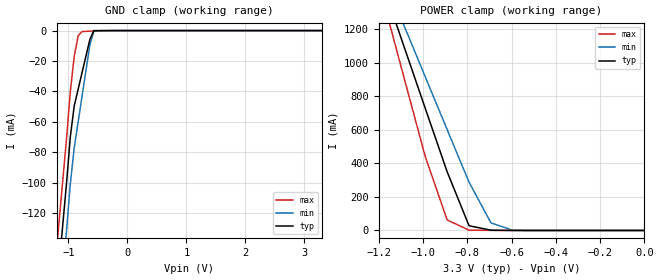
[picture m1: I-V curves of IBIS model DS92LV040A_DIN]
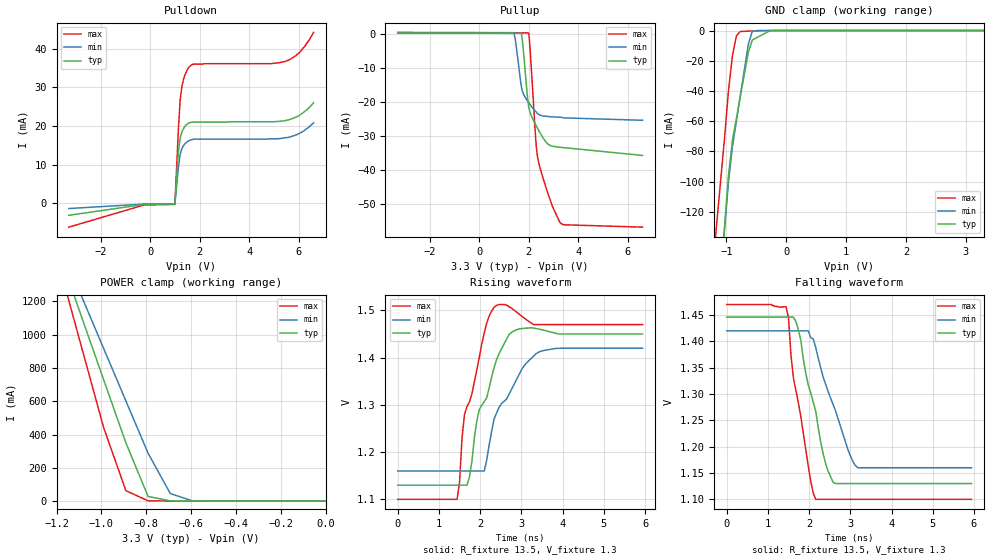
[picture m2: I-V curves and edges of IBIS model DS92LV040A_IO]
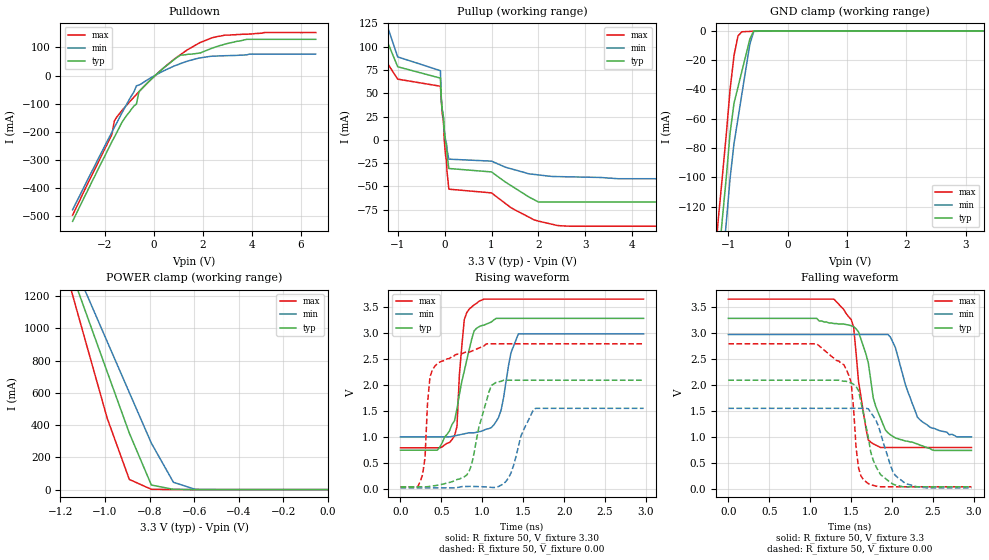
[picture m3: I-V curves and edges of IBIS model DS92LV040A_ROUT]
|   National Semiconductor Corporation
|   IBIS Model of DS92LV040A
|   4 Channel Bus LVDS Transceiver
|   44 Lead LLP Package
[IBIS Ver]   3.2
[Comment Char]   |_char
[File name]   ds92lv040atlqa.ibs
[File Rev]   2.2
[Date]   08/23/04
[Source]
SPICE to IBIS Translation
[Notes]
Created by Tim Coyle
Rev2.1 adjusted IOM and IOP rise fall tables for monotonicity--milt
Rev2.2 Updated Power clamp tables, C-comp, Pin, Package, and Ramp;
   New DS92LV040A_IO model; dglisic
[Disclaimer]
(C) Copyright National Semiconductor Corporation 2002
   All rights reserved
   National Semiconductor Corporation hereby grants
the user of this IBIS model a non-exclusive, nontransferable
license to use this IBIS model under the following terms.
Before using this IBIS model, the user should read this
license.  If the user does not accept these terms,  the
IBIS model should be returned to National within 30 days.
   The user is granted this license only to use the
IBIS model and is not granted rights to sell, load, rent,
lease or license the IBIS model in whole or in part, or in
modified form to anyone other than user. User may modify
the IBIS model to suit its specific applications but rights
to derivative works and such modifications shall belong to
National.
   This IBIS model is provided on an "AS IS" basis and
National makes absolutely no warranty with respect to the
information contained herein.NATIONAL DISCLAIMS AND CUSTOMER
WAIVES ALL WARRANTIES, EXPRESS OR IMPLIED, INCLUDING
WARRANTIES OF MERCHANTABILITY OR FITNESS FOR A PARTICULAR
PURPOSE. The entire risk as to quality and performance is
with the Customer. ACCORDINGLY, IN NO EVENT SHALL THE
COMPANY BE LIABLE FOR ANY DAMAGES, WHETHER IN CONTRACT OR
TORT,INCLUDING ANY LOST PROFITS OR OTHER INCIDENTAL,
CONSEQUENTIAL, EXEMPLARY, OR PUNITIVE DAMAGES ARISING OUT
OF THE USE OR APPLICATION OF THE IBIS model provided in
this package.Further, National reserves the right to make
changes without notice to any product herein to improve
reliability, function, or design. National does not convey
any license under patent rights or any other intellectual
property rights, including those of third parties.
   National is not obligated to provide maintenance or support
for the licensed IBIS model.
Contact National at ATTN:INTERFACE APPLICATIONS/IBIS MODELS.
5 Foden Road, M/S 03-03, South Porltand, ME 04106
(207) 541-6031
[Copyright]
(c) Copyright 2002 National Semiconductor Corp.
[Component]   DS92LV040ATLQA
Si_location Pin
Timing_location Pin
[Manufacturer]   National Semiconductor Corp.
[Package]
|   TYP   MIN   MAX
R_pkg   0.194   0.174   0.249
L_pkg   1.88n   1.46n   2.21n
C_pkg   0.084p   0.063p   0.111p
[Pin]   signal_name   model_name   R_pin   L_pin   C_pin
1   NC   NC   0.239   2.15n   0.094p
2   NC   NC   0.223   1.96n   0.074p
3   VCC   POWER   0.210   1.83n   0.071p
4   GND   GND   0.214   1.78n   0.102p
5   RE2*   DS92LV040A_CONTROL  0.222   1.80n   0.103p
6   VCC   POWER   0.200   1.73n   0.072p
7   AVCC   POWER   0.194   1.67n   0.073p
8   DE2   DS92LV040A_CONTROL  0.194   1.66n   0.072p
9   AGND   GND   0.197   1.70n   0.070p
10   VCC   POWER   0.209   1.81n   0.071p
11   NC   NC   0.223   1.96n   0.074p
12   NC   NC   0.237   2.13n   0.093p
13   DO4-_RIN4-   DS92LV040A_IO   0.205   1.78n   0.084p
14   DO4+_RIN4+   DS92LV040A_IO   0.189   1.61n   0.065p
15   DO3-_RIN3-   DS92LV040A_IO   0.190   1.54n   0.091p
16   DO3+_RIN3+   DS92LV040A_IO   0.189   1.51n   0.086p
17   AGND   GND   0.175   1.46n   0.063p
18   DO2-_RIN2-   DS92LV040A_IO   0.174   1.46n   0.064p
19   DO2+_RIN2+   DS92LV040A_IO   0.185   1.55n   0.063p
20   DO1-_RIN1-   DS92LV040A_IO   0.215   1.70n   0.075p
21   DO1+_RIN1+   DS92LV040A_IO   0.230   1.75n   0.079p
22   AVCC   POWER   0.242   1.89n   0.093p
23   NC   NC   0.249   2.16n   0.111p
24   NC   NC   0.231   1.95n   0.089p
25   AGND   GND   0.214   1.81n   0.084p
26   DE1   DS92LV040A_CONTROL  0.203   1.74n   0.066p
27   AVCC   POWER   0.202   1.68n   0.082p
28   GND   GND   0.207   1.69n   0.081p
29   RE1*   DS92LV040A_CONTROL  0.207   1.70n   0.082p
30   VCC   POWER   0.214   1.77n   0.080p
31   GND   GND   0.229   1.87n   0.095p
32   NC   NC   0.231   1.91n   0.082p
33   NC   NC   0.234   1.96n   0.083p
34   NC   NC   0.248   2.21n   0.090p
35   DIN1   DS92LV040A_DIN   0.217   1.83n   0.098p
36   RO1   DS92LV040A_ROUT   0.204   1.70n   0.080p
37   DIN2   DS92LV040A_DIN   0.196   1.65n   0.080p
38   RO2   DS92LV040A_ROUT   0.194   1.54n   0.076p
39   GND   GND   0.175   1.46n   0.063p
40   DIN3   DS92LV040A_DIN   0.182   1.48n   0.078p
41   RO3   DS92LV040A_ROUT   0.184   1.50n   0.076p
42   DIN4   DS92LV040A_DIN   0.187   1.58n   0.063p
43   RO4   DS92LV040A_ROUT   0.203   1.68n   0.082p
44   NC   NC   0.216   1.80n   0.099p
[Diff Pin] inv_pin   vdiff   tdelay_typ   tdelay_min   tdelay_max
| The '+' pin is Diff_pin and the '-' pin is the inv_pin
| Receiver Vth = +/-100mV
14   13   0.1   0   0   0
16   15   0.1   0   0   0
19   18   0.1   0   0   0
21   20   0.1   0   0   0
| Models and submodels in the file (4): DS92LV040A_DIN (Input), DS92LV040A_IO (I/O), DS92LV040A_ROUT (3-state), DS92LV040A_CONTROL (Input)
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[Model]   DS92LV040A_DIN
Model_type Input
Vinh=2.0
Vinl=0.8
C_comp   3.834p   3.834p   3.834p
[Model Spec]
S_overshoot_high   3.6   3.3   3.9
S_overshoot_low   -0.3   -0.3   -0.3
[Temperature Range] 25   85   -40
[Voltage Range]   3.3   3.00   3.60
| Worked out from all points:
|   GND clamp passes 1 mA (typ) near -0.58 V on its own axis
|   POWER clamp passes 1 mA (typ) near -0.65 V on its own axis
[GND Clamp]
|V(groundclamp)   I(typ)   I(min)   I(max)
-3.3V     -1.29A     -1.28A     -1.31A
-1.17V    -161mA     -192mA     -131mA
-1.1V     -130mA     -161mA     -101mA
-1.03V    -100mA     -131mA     -70.6mA
-967mV    -70mA      -101mA     -40.4mA
-900mV    -49.4mA    -76.9mA    -16.8mA
-833mV    -38.4mA    -59.9mA    -3.44mA
-767mV    -27.5mA    -42.9mA    -643uA
-633mV    -5.52mA    -8.94mA    -387uA
-567mV    -32.1uA    -395uA     -259uA
3.3V      456pA      883pA      215pA
[POWER Clamp]
|Vtable   I(typ)   I(min)   I(max)
-3.267V   9.584A     8.291A     11.75A
-1.188V   1.491A     1.55A      1.416A
-1.089V   1.11A      1.233A     928.2mA
-990mV    729.5mA    917.3mA    441.9mA
-891mV    350.5mA    602.3mA    63.05mA
-792mV    28.24mA    288.1mA    1.817mA
-693mV    1.617mA    45.27mA    453.5uA
-594mV    118.9uA    1.221mA    66.77uA
0V        857.1pA    1.83nA     132.3pA
[Model]   DS92LV040A_IO
Model_type I/O
Polarity Non-Inverting
Vref=1.30
Vmeas=1.30
Rref=13.5   | 27 Ohms Across Outputs OUTP and OUTM
Cref=10p
Vinl = -0.1
Vinh =  0.1
C_comp   5p   5p   5p
[Model Spec]
S_overshoot_high   3.6   3.3   3.9
S_overshoot_low   -0.3   -0.3   -0.3
[Temperature Range] 25   85   -40
[Voltage Range]   3.3   3.00   3.60
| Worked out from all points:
|   slope of the pulldown table from 0 to 0.495 V, typ, clamps not added: 15.5 kohm
|   GND clamp passes 1 mA (typ) near -0.31 V on its own axis
|   POWER clamp passes 1 mA (typ) near -0.65 V on its own axis
|   falling waveform, R_fixture 13.5, V_fixture 1.3: 20-80 % time 492ps typ, 648ps min, 417ps max; typ from 1.45 V to 1.13 V
|   rising waveform, R_fixture 13.5, V_fixture 1.3: 20-80 % time 547ps typ, 754ps min, 444ps max; typ from 1.13 V to 1.45 V
[Pullup]
|Vtable   I(typ)   I(min)   I(max)
-3.3V     193uA      113uA      358uA
1.4V      120uA      64.1uA     244uA
1.45V     116uA      -1.52mA    237uA
1.7V      92.1uA     -15.6mA    205uA
1.75V     -2.58mA    -17.1mA    199uA
2V        -21.7mA    -20.3mA    118uA
2.05V     -23.1mA    -20.8mA    -4.23mA
2.3V      -27mA      -23mA      -32.9mA
2.35V     -27.7mA    -23.4mA    -36mA
2.75V     -32.2mA    -24.3mA    -46.3mA
3.25V     -33.3mA    -24.5mA    -55.2mA
6.6V      -35.7mA    -25.4mA    -56.7mA
[Pulldown]
|V(pulldown)   I(typ)   I(min)   I(max)
-3.3V     -3.08mA    -1.33mA    -6.14mA
-287mV    -259uA     -168uA     -432uA
991mV     -153uA     -100uA     -264uA
1.133V    13.2mA     9.34mA     19.1mA
1.204V    16.9mA     12.7mA     26.7mA
1.275V    18.5mA     14.2mA     30.3mA
1.346V    19.4mA     15mA       32.2mA
1.488V    20.5mA     15.9mA     34.5mA
1.63V     20.9mA     16.4mA     35.6mA
5.464V    21.4mA     17mA       36.7mA
6.032V    22.8mA     18.1mA     39mA
6.6V      26mA       20.8mA     44.2mA
[GND Clamp]
|V(groundclamp)   I(typ)   I(min)   I(max)
-3.3V     -1.36A     -1.28A     -1.31A
-1.17V    -195mA     -192mA     -131mA
-1.1V     -162mA     -161mA     -101mA
-1.03V    -129mA     -131mA     -70.6mA
-967mV    -96.5mA    -101mA     -40.4mA
-900mV    -72.8mA    -76.9mA    -16.8mA
-833mV    -58.1mA    -59.9mA    -3.44mA
-767mV    -43.5mA    -42.9mA    -643uA
-633mV    -14.3mA    -8.94mA    -387uA
-567mV    -6.25mA    -395uA     -259uA
-233mV    -5.33uA    -194nA     -1.26uA
3.3V      984pA      883pA      215pA
[POWER Clamp]
|Vtable   I(typ)   I(min)   I(max)
-3.267V   9.584A     8.291A     11.75A
-1.188V   1.491A     1.55A      1.416A
-1.089V   1.11A      1.233A     928.2mA
-990mV    729.5mA    917.3mA    441.9mA
-891mV    350.5mA    602.3mA    63.05mA
-792mV    28.24mA    288.1mA    1.817mA
-693mV    1.617mA    45.27mA    453.5uA
-594mV    118.9uA    1.221mA    66.77uA
0V        857.1pA    1.83nA     132.3pA
|IO
[Ramp]
dV/dt_r   192mV/.647ns   156mV/.940ns   222mV/.474ns
dV/dt_f   192mv/.466ns   156mv/.577ns   222mv/.384ns
R_load=13.5
|IO
[Falling Waveform]
R_fixture=13.5
V_fixture=1.3
V_fixture_min=1.3
V_fixture_max=1.3
0s        1.446V     1.42V      1.47V
1.44ns    1.446V     1.42V      1.466V
1.5ns     1.446V     1.42V      1.445V
1.68ns    1.438V     1.42V      1.307V
1.98ns    1.317V     1.42V      1.163V
2.16ns    1.267V     1.389V     1.1V
2.34ns    1.187V     1.332V     1.1V
2.58ns    1.133V     1.28V      1.1V
3.18ns    1.13V      1.16V      1.1V
5.94ns    1.13V      1.16V      1.1V
|IO
[Rising Waveform]
R_fixture=13.5
V_fixture=1.3
V_fixture_min=1.3
V_fixture_max=1.3
0s        1.13V      1.16V      1.1V
1.44ns    1.13V      1.16V      1.1V
1.62ns    1.13V      1.16V      1.28V
1.74ns    1.147V     1.16V      1.306V
1.98ns    1.29V      1.16V      1.401V
2.1ns     1.307V     1.16V      1.452V
2.4ns     1.396V     1.283V     1.511V
2.76ns    1.453V     1.333V     1.505V
3.42ns    1.46V      1.412V     1.47V
5.94ns    1.45V      1.42V      1.47V
[Model]   DS92LV040A_ROUT
Model_type 3-state
Polarity Non-Inverting
Vref=0.0
Vmeas=1.65
Cref=15p
C_comp   5p   5p   5p
[Temperature Range] 25   85   -40
[Voltage Range]   3.3   3.00   3.60
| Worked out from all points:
|   slope of the pulldown table from 0 to 0.495 V, typ, clamps not added: 12.9 ohm
|   slope of the pullup table from 0 to 0.495 V, typ, clamps not added: 12.4 ohm
|   GND clamp passes 1 mA (typ) near -0.58 V on its own axis
|   POWER clamp passes 1 mA (typ) near -0.65 V on its own axis
|   falling waveform, R_fixture 50, V_fixture 3.3: 20-80 % time 245ps typ, 241ps min, 128ps max; typ from 3.29 V to 0.75 V
|   rising waveform, R_fixture 50, V_fixture 3.30: 20-80 % time 219ps typ, 142ps min, 74.2ps max; typ from 0.755 V to 3.29 V
|   falling waveform, R_fixture 50, V_fixture 0.00: 20-80 % time 179ps typ, 188ps min, 120ps max; typ from 2.1 V to 0.05 V
|   rising waveform, R_fixture 50, V_fixture 0.00: 20-80 % time 183ps typ, 184ps min, 80.6ps max; typ from 0.05 V to 2.1 V
[Pullup]
|Vtable   I(typ)   I(min)   I(max)
-3.3V     539mA      529mA      495mA
-1.4V     137mA      151mA      159mA
-1.3V     120mA      135mA      89.1mA
-1.2V     103mA      119mA      80.9mA
-1V       78.5mA     89.1mA     65.2mA
-90mV     66.3mA     74.3mA     57.6mA
-70mV     42mA       44.5mA     42.5mA
-10mV     12mA       10.6mA     920uA
90mV      -30.7mA    -20.7mA    -52.9mA
1V        -34.4mA    -22.8mA    -56.9mA
2V        -66.7mA    -37.6mA    -87.2mA
6.6V      -66.7mA    -41.7mA    -92.7mA
[Pulldown]
|V(pulldown)   I(typ)   I(min)   I(max)
-3.3V     -518mA     -477mA     -496mA
-1.7V     -235mA     -201mA     -210mA
-1.6V     -219mA     -184mA     -161mA
-1.2V     -154mA     -118mA     -115mA
-700mV    -101mA     -36.2mA    -66.9mA
-600mV    -57.4mA    -33.7mA    -57.4mA
900mV     61.5mA     36.3mA     62.5mA
1.1V      72.9mA     42.8mA     74.9mA
1.9V      80.4mA     63mA       118mA
2.9V      112mA      70.7mA     144mA
3.8V      129mA      73.8mA     147mA
6.6V      129mA      76.6mA     153mA
[GND Clamp]
|V(groundclamp)   I(typ)   I(min)   I(max)
-3.3V     -1.29A     -1.28A     -1.31A
-1.17V    -161mA     -192mA     -131mA
-1.1V     -130mA     -161mA     -101mA
-1.03V    -100mA     -131mA     -70.6mA
-967mV    -70mA      -101mA     -40.4mA
-900mV    -49.4mA    -76.9mA    -16.8mA
-833mV    -38.4mA    -59.9mA    -3.44mA
-767mV    -27.5mA    -42.9mA    -643uA
-633mV    -5.52mA    -8.94mA    -387uA
-567mV    -32.1uA    -395uA     -259uA
3.3V      456pA      883pA      215pA
[POWER Clamp]
|Vtable   I(typ)   I(min)   I(max)
-3.267V   9.584A     8.291A     11.75A
-1.188V   1.491A     1.55A      1.416A
-1.089V   1.11A      1.233A     928.2mA
-990mV    729.5mA    917.3mA    441.9mA
-891mV    350.5mA    602.3mA    63.05mA
-792mV    28.24mA    288.1mA    1.817mA
-693mV    1.617mA    45.27mA    453.5uA
-594mV    118.9uA    1.221mA    66.77uA
0V        857.1pA    1.83nA     132.3pA
[Ramp]
dV/dt_r   2.0V/1ns   1.8V/2ns   2.2V/.8ns
dV/dt_f   2.0V/1ns   1.8V/2ns   2.2V/.8ns
R_load=50
[Falling Waveform]
R_fixture=50
V_fixture=3.3
V_fixture_min=3.00
V_fixture_max=3.60
0s        3.29V      2.98V      3.66V
1.29ns    3.19V      2.98V      3.66V
1.53ns    3.13V      2.98V      3.13V
1.59ns    3.03V      2.98V      2.08V
1.71ns    2.43V      2.98V      950mV
1.77ns    1.76V      2.98V      877mV
1.95ns    1.09V      2.98V      806mV
2.04ns    991mV      2.73V      806mV
2.31ns    873mV      1.39V      806mV
2.97ns    750mV      1.01V      806mV
[Rising Waveform]
R_fixture=50
V_fixture=3.30
V_fixture_min=3.00
V_fixture_max=3.60
0s        755mV      1.01V      801mV
450ps     755mV      1.01V      801mV
660ps     1.32V      1.03V      1.03V
690ps     1.55V      1.04V      1.21V
720ps     1.83V      1.05V      2.21V
780ps     2.28V      1.07V      3.27V
960ps     3.13V      1.11V      3.62V
1.2ns     3.29V      1.39V      3.66V
1.44ns    3.29V      2.99V      3.66V
2.97ns    3.29V      2.99V      3.66V
[Falling Waveform]
R_fixture=50
V_fixture=0.00
V_fixture_min=0.00
V_fixture_max=0.00
0s        2.1V       1.56V      2.8V
1.08ns    2.1V       1.56V      2.8V
1.41ns    2.08V      1.56V      2.4V
1.5ns     2.05V      1.56V      2.06V
1.59ns    1.9V       1.56V      415mV
1.71ns    996mV      1.55V      111mV
1.86ns    285mV      1.08V      50.7mV
2.01ns    102mV      339mV      50.7mV
2.13ns    50.4mV     155mV      50.7mV
2.97ns    50.4mV     30mV       50.7mV
[Rising Waveform]
R_fixture=50
V_fixture=0.00
V_fixture_min=0.00
V_fixture_max=0.00
0s        50.3mV     30.2mV     50.5mV
270ps     50.3mV     30.2mV     284mV
300ps     50.3mV     30.2mV     615mV
360ps     59.3mV     30.2mV     2.16V
480ps     88.6mV     30.2mV     2.45V
840ps     355mV      58mV       2.64V
1.17ns    2.06V      41.8mV     2.8V
1.35ns    2.1V       317mV      2.8V
1.65ns    2.1V       1.56V      2.8V
2.97ns    2.1V       1.56V      2.8V
